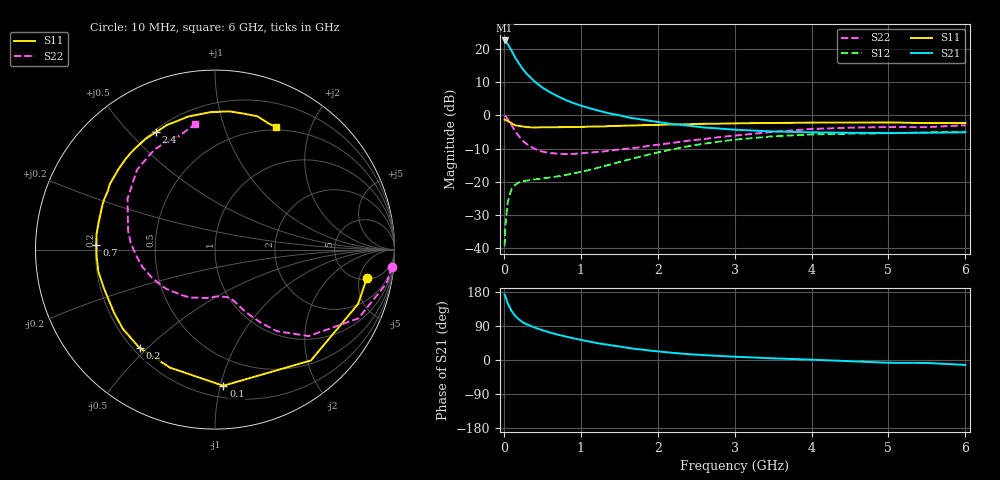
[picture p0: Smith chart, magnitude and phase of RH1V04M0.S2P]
! SIEMENS Small Signal Semiconductors
! BFR106
! Si NPN RF Bipolar Junction Transistor in SOT23
! VCE = 1 V  IC = 4 mA
! Common Emitter S-Parameters:  August  1996
# GHz  S  MA  R  50
!  f  S11  S21  S12  S22
! GHz  MAG  ANG  MAG  ANG  MAG  ANG  MAG  ANG
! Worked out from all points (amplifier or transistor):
!   36 points, 10 MHz to 6 GHz, reference 50 ohm
!   highest |S21| = 22.5 dB at 10 MHz (marker M1)
!   |S21| within 3 dB of that: start of sweep to 98.69 MHz
!   unconditionally stable (mu >= 1): 637.7 MHz to end of sweep
!   at 250 MHz: K = 0.46, MSG = 16.8 dB, |S12| = -19.8 dB
!   at 1.4 GHz: K = 1.22, MAG = 4.8 dB, |S12| = -14.7 dB
!   at 6 GHz: K = 1.03, MAG = -1.1 dB, |S12| = -4.9 dB
!   S11 on the Smith chart (normalised r, x): 10 MHz: 5.31, -6.49; 100 MHz: 0.28, -1.02; 200 MHz: 0.23, -0.47; 700 MHz: 0.20, +0.02; 2.4 GHz: 0.21, +0.60; 6 GHz: 0.47, +1.51
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0.01  0.8607 -10.6  13.3 172.9  0.0108 85.7  0.9901 -5.5
0.02  0.8529 -20.8  13.11 167.4  0.0214 79.6  0.9743 -11.1
0.05  0.8169 -49.1  11.74 150.0  0.0492 64.3  0.8861 -25.6
0.1  0.7599 -86.5  9.362 129.7  0.0779 48.1  0.7107 -42.7
0.15  0.7039 -110.8  7.279 115.5  0.0911 38.5  0.5696 -52.9
0.2  0.6908 -127.5  5.911 106.5  0.0984 33.6  0.4777 -58.1
0.25  0.677 -139.3  4.893 99.1  0.1021 30.8  0.4085 -62.3
0.3  0.6639 -147.8  4.165 94.1  0.1047 29.8  0.3673 -65.1
0.4  0.6552 -160.6  3.214 85.7  0.1088 29.2  0.3127 -69.0
0.5  0.6614 -169.3  2.612 78.7  0.1124 30.5  0.2846 -72.5
0.6  0.6602 -176.5  2.215 72.5  0.1163 32.6  0.271 -76.7
0.7  0.6616 177.6  1.932 67.0  0.121 35.3  0.2654 -81.4
0.9  0.6647 167.7  1.53 57.5  0.1336 40.6  0.2624 -90.1
1.1  0.6745 158.6  1.289 49.1  0.1496 45.4  0.2747 -100.5
1.3  0.6806 151.2  1.118 41.7  0.1718 48.9  0.286 -110.9
1.6  0.6987 140.9  0.938 32.5  0.2124 51.4  0.3148 -126.4
2.2  0.7278 122.3  0.735 18.8  0.3099 47.7  0.3854 -156.2
2.4  0.7326 116.6  0.698 15.4  0.3431 44.8  0.4154 -166.4
3.5  0.7662 91.8  0.571 4.4  0.4832 24.7  0.5635 149.9
4.5  0.7744 77.7  0.545 -3.2  0.5296 7.8  0.6512 121.4
5.5  0.7643 67.3  0.546 -7.8  0.5523 -2.1  0.663 107.9
6  0.7622 63.5  0.555 -13.0  0.5677 -8.8  0.7076 99.0
